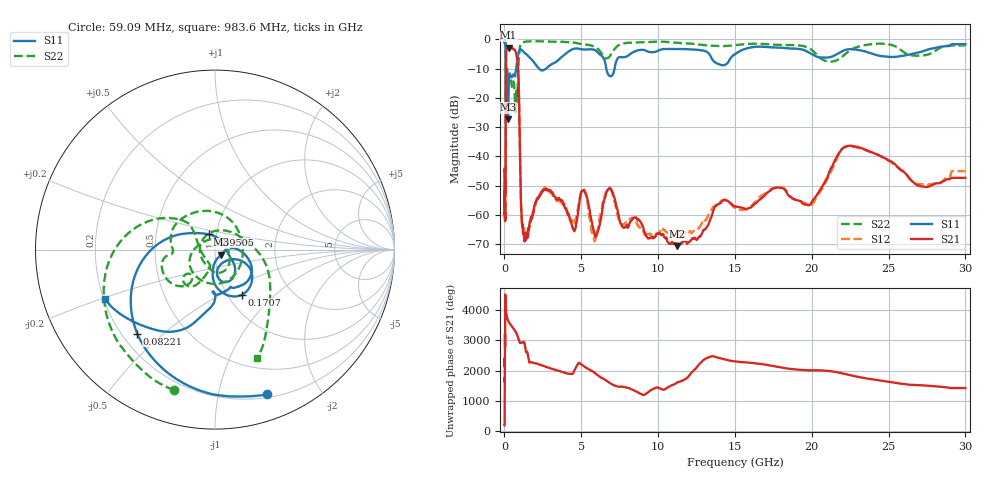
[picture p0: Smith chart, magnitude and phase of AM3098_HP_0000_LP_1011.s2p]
! Date/Time: Thu, Feb 28, 2019 8:31 AM
! Network Analyzer: Agilent Technologies E8364B Rev: A.07.50.67
! Sweep from 0.010 to 30.000 GHz, 1601 Points, Sweep Type: LOG
! Power Supply: 5.023 V, 0.002 A
# Hz S DB R 50
!freq MagS11 AngS11 MagS21 AngS21 MagS12 AngS12 MagS22 AngS22
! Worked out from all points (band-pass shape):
!   1601 points, 10 MHz to 30 GHz, reference 50 ohm
!   highest |S21| = -2.80 dB at 266.5 MHz (marker M1); lowest = -70.7 dB at 11.25 GHz (marker M2)
!   |S21| within 3 dB of the highest: 104.6 MHz to 806.9 MHz (702.3 MHz wide, 154 % of centre)
!   lowest |S11| = -27.3 dB at 232.8 MHz (marker M3), VSWR 1.09, Z = 53.3 - j3 ohm
!   |S11| at or under -10 dB: 90.38 MHz to 756.6 MHz (666.3 MHz wide, 157 % of centre); 2.27 GHz to 2.709 GHz (439.1 MHz wide, 17.6 % of centre); 6.629 GHz to 7.168 GHz (538.8 MHz wide, 7.81 % of centre)
!   |S22| runs from -24.9 to -0.6 dB; largest |S21 - S12| = 0.01
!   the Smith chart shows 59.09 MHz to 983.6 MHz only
!   S11 on the Smith chart (normalised r, x): 59.09 MHz: 0.23, -1.40; 82.21 MHz: 0.26, -0.41; 95.05 MHz: 0.92, +0.16; 170.7 MHz: 1.16, -0.64; 983.6 MHz: 0.21, -0.21
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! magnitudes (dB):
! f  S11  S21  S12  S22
! 10 MHz  -0.3  -44.2  -47.7  -0.6
! 38.04 MHz  -0.5  -61.3  -59.2  -1.0
! 59.09 MHz  -1.3  -49.3  -49.9  -1.8
! 82.21 MHz  -3.9  -32.2  -32.2  -4.4
! 95.05 MHz  -20.8  -9.9  -9.8  -22.4
! 144.7 MHz  -14.3  -3.5  -3.4  -12.7
! 170.7 MHz  -10.7  -3.4  -3.3  -10.0
! 232.8 MHz  -27.3  -2.9  -2.9  -12.4
! 266.5 MHz  -17.2  -2.8  -2.8  -12.6
! 550.5 MHz  -12.2  -3.2  -3.1  -14.6
! 850.8 MHz  -6.6  -7.6  -7.6  -19.1
! 983.6 MHz  -3.5  -31.0  -31.0  -3.7
! 1.104 GHz  -3.5  -59.0  -59.5  -1.3
! 1.257 GHz  -4.3  -67.1  -65.6  -0.9
! 2.084 GHz  -8.9  -55.2  -54.8  -0.6
! 5.9 GHz  -3.7  -67.3  -68.7  -2.6
! 6.855 GHz  -12.5  -50.8  -50.9  -5.7
! 7.926 GHz  -5.9  -63.7  -62.6  -1.2
! 11.25 GHz  -3.3  -70.7  -67.2  -1.2
! 19.8 GHz  -4.4  -56.7  -56.7  -3.0
! 22.56 GHz  -3.4  -36.3  -36.5  -3.5
! 30 GHz  -1.6  -47.4  -45.1  -2.1
